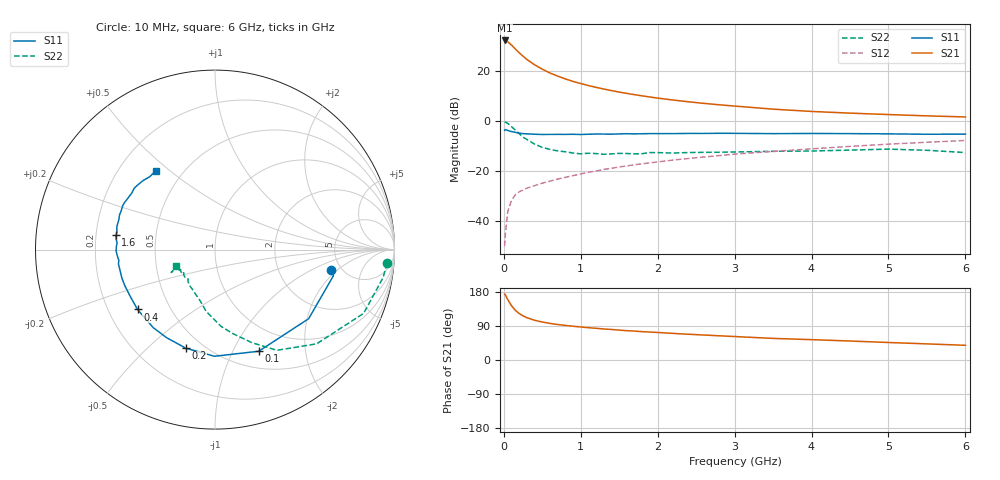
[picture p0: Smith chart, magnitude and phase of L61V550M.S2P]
!  INFINEON TECHNOLOGIES Small Signal Semiconductors
! BFR380L3 , Si-NPN RF-Transistor in TSLP-3-1
!  Vce=1.5 V,  Ic=50 mA
! Common Emitter S-Parameters:  07. March 2005
#  GHz  S  MA  R  50
! f  S11  S21  S12  S22
! GHz  Mag  Ang  Mag  Ang  Mag  Ang  Mag  Ang
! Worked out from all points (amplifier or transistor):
!   36 points, 10 MHz to 6 GHz, reference 50 ohm
!   highest |S21| = 32.1 dB at 10 MHz (marker M1)
!   |S21| within 3 dB of that: start of sweep to 137.3 MHz
!   unconditionally stable (mu >= 1): 1.531 GHz to 4.976 GHz
!   at 250 MHz: K = 0.47, MSG = 26.7 dB, |S12| = -27.5 dB
!   at 1.4 GHz: K = 1.00, MSG = 15.5 dB, |S12| = -18.8 dB
!   at 6 GHz: K = 0.99, MSG = 4.7 dB, |S12| = -7.7 dB
!   S11 on the Smith chart (normalised r, x): 10 MHz: 4.09, -1.64; 100 MHz: 0.69, -1.27; 200 MHz: 0.41, -0.66; 400 MHz: 0.33, -0.31; 1.6 GHz: 0.28, +0.07; 6 GHz: 0.36, +0.45
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0.01  0.6544 -10.1  40.39 174.1  0.0032 73.9  0.9618 -4.5
0.02  0.6759 -12.4  40.02 171.9  0.0056 80.4  0.9492 -9.5
0.05  0.6485 -36.4  38.02 159.6  0.0154 75.0  0.9012 -23.2
0.1  0.6166 -66.7  32.67 143.2  0.0264 62.6  0.7725 -42.8
0.15  0.5943 -90.3  27.33 131.0  0.0339 56.7  0.6587 -58.4
0.2  0.5728 -106.5  22.91 122.6  0.0388 53.8  0.5585 -68.3
0.25  0.5599 -118.8  19.57 116.5  0.0422 50.9  0.4765 -78.3
0.3  0.5545 -128.4  16.87 111.6  0.0459 50.7  0.429 -85.5
0.4  0.5455 -142.3  13.21 104.8  0.0515 51.6  0.3469 -98.3
0.5  0.5393 -151.5  10.8 100.2  0.0577 53.1  0.2981 -105.9
0.6  0.5411 -158.0  9.058 96.6  0.0634 55.1  0.2719 -113.2
0.7  0.5424 -162.8  7.85 93.7  0.0697 57.1  0.2533 -120.3
0.9  0.544 -171.6  6.151 89.1  0.0816 59.7  0.2302 -131.0
1.1  0.5459 -176.6  5.091 85.2  0.0953 61.6  0.2282 -136.0
1.3  0.5494 177.9  4.345 81.8  0.1086 62.6  0.2169 -143.5
1.6  0.5585 171.7  3.549 77.4  0.1274 63.6  0.2253 -149.3
2.2  0.5611 162.7  2.624 70.2  0.1666 64.5  0.2299 -151.0
2.8  0.5696 154.4  2.107 63.9  0.2046 64.3  0.2387 -155.7
3.5  0.5605 146.1  1.725 57.0  0.2475 62.2  0.2493 -154.3
4.5  0.5611 139.9  1.437 50.1  0.3124 60.2  0.2632 -153.3
5.5  0.545 131.8  1.268 42.5  0.3773 56.1  0.261 -153.4
6  0.5489 126.8  1.206 38.8  0.4098 53.8  0.2352 -157.1
